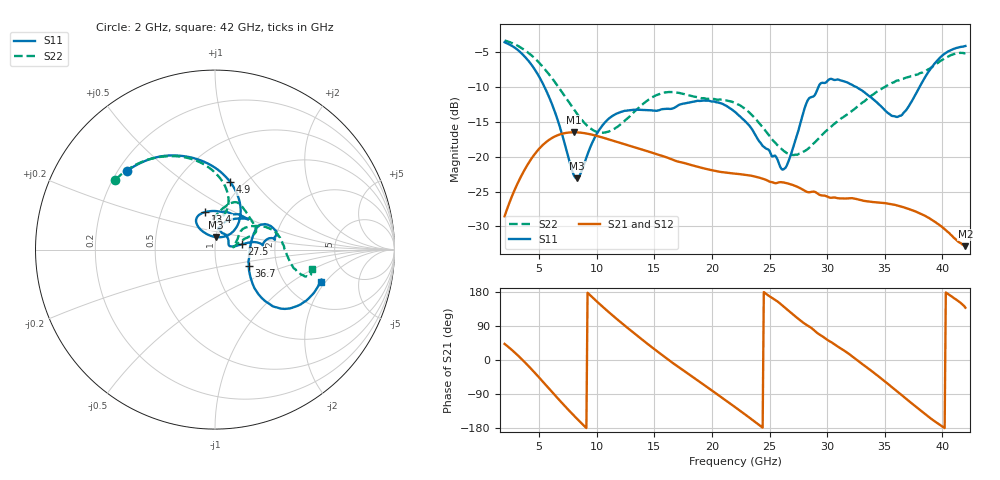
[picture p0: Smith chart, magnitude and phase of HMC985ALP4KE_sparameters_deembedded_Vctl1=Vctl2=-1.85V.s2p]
!s2p File: Measurements: S11, S21, S12, S22
# GHz S dB R 50.0
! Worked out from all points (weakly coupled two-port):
!   401 points, 2 GHz to 42 GHz, reference 50 ohm
!   highest |S21| = -16.51 dB at 8 GHz (marker M1); lowest = -32.8 dB at 42 GHz (marker M2)
!   lowest |S11| = -23.1 dB at 8.3 GHz (marker M3), VSWR 1.15, Z = 50 + j7.01 ohm
!   |S11| at or under -10 dB: 5.453 GHz to 29.25 GHz (23.8 GHz wide, 137 % of centre); 32.48 GHz to 38.03 GHz (5.55 GHz wide, 15.7 % of centre)
!   |S22| runs from -19.8 to -3.4 dB; largest |S21 - S12| = 0.00015
!   S11 on the Smith chart (normalised r, x): 2 GHz: 0.23, +0.36; 4.9 GHz: 0.87, +0.77; 13.4 GHz: 0.82, +0.36; 27.5 GHz: 1.35, +0.08; 36.7 GHz: 1.44, -0.27; 42 GHz: 3.12, -1.80
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2  -3.63 138.4  -28.54 42.5  -28.54 42.5  -3.37 144.9
3.4  -5.11 109.8  -22.92 4.8  -22.92 4.8  -4.38 121.4
4.9  -8.28 77.3  -19.05 -43.0  -19.06 -43.0  -6.39 97.4
6.1  -12.43 53.6  -17.35 -83.8  -17.35 -83.8  -8.75 81.8
8  -22.61 68.7  -16.51 -146.2  -16.52 -146.2  -13.21 73.9
8.3  -23.11 86.2  -16.53 -155.5  -16.53 -155.5  -13.90 75.2
8.7  -22.00 106.4  -16.59 -167.7  -16.59 -167.7  -14.74 78.0
10.7  -15.12 125.5  -17.36 135.4  -17.36 135.4  -16.55 95.2
13.4  -13.29 104.8  -18.73 66.8  -18.73 66.8  -13.36 83.2
15.4  -13.37 79.0  -19.77 19.4  -19.77 19.4  -11.05 69.6
18.9  -12.03 43.4  -21.51 -56.9  -21.52 -56.9  -11.55 44.0
22  -13.60 55.5  -22.44 -124.2  -22.45 -124.2  -12.32 22.4
24.5  -18.60 81.2  -23.21 179.2  -23.21 179.2  -15.99 18.5
26.1  -21.85 20.2  -23.67 144.1  -23.68 144.1  -19.00 10.3
27.5  -16.29 11.0  -24.40 108.6  -24.39 108.5  -19.64 8.3
28.7  -11.44 5.4  -25.03 82.9  -25.04 82.9  -18.32 17.8
31.1  -9.06 17.7  -25.98 32.2  -25.99 32.2  -14.69 36.2
33.3  -10.88 28.6  -26.36 -16.2  -26.37 -16.2  -12.00 31.3
35.4  -13.90 8.5  -26.76 -66.2  -26.77 -66.2  -9.68 20.7
36.7  -13.61 -25.2  -27.29 -98.4  -27.30 -98.5  -8.79 11.9
39.6  -6.18 -42.0  -29.62 -167.4  -29.62 -167.5  -6.59 -14.5
42  -4.17 -16.7  -32.82 137.9  -32.80 137.8  -5.18 -11.5
